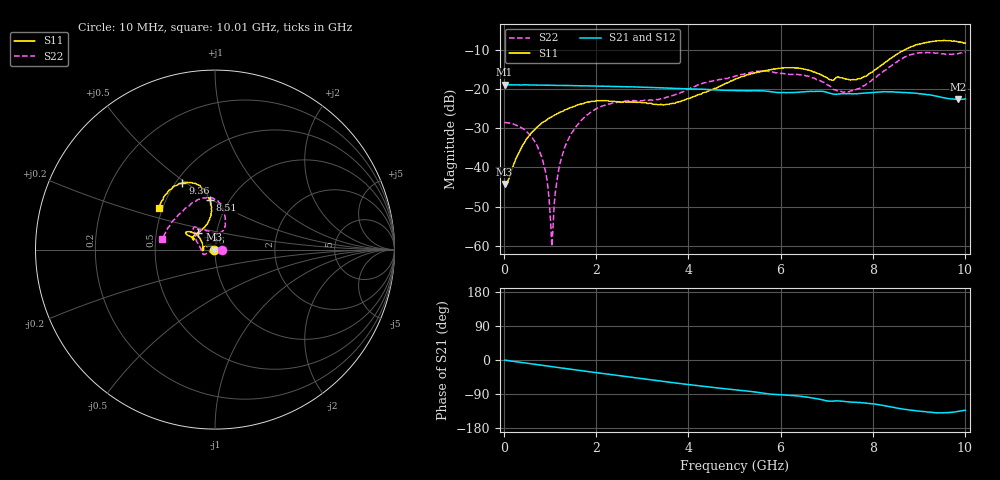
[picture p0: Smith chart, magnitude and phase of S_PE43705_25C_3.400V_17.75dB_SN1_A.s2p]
! Device ID: PE43705
! Serial: 1
! Insertion: A
! Impedance: 50 ohm
! Temp: 25C
! VDD: 3.400V
! Attenuation Step: 17.75dB
#  Hz  S  RI  R  50
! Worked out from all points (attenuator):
!   401 points, 10 MHz to 10.01 GHz, reference 50 ohm
!   highest |S21| = -18.83 dB at 10 MHz (marker M1); lowest = -22.6 dB at 9.86 GHz (marker M2)
!   lowest |S11| = -44.2 dB at 10 MHz (marker M3), VSWR 1.01, Z = 49.4 + j0.0483 ohm
!   |S11| at or under -10 dB: start of sweep to 8.677 GHz
!   |S22| runs from -60.1 to -10.4 dB; largest |S21 - S12| = 0.0014
!   S11 on the Smith chart (normalised r, x): 10 MHz: 0.99, +0.00; 7.46 GHz: 0.81, +0.16; 8.51 GHz: 0.82, +0.48; 9.36 GHz: 0.54, +0.48; 10.01 GHz: 0.48, +0.26
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1e7  -0.00614 0.000489  0.1144 -0.000478  0.1145 -0.000386  0.0375 -7.58e-06
4.1e8  -0.0103 0.0165  0.1132 -0.0135  0.1129 -0.0141  0.0309 0.00518
7.1e8  -0.0211 0.0248  0.1106 -0.0238  0.1106 -0.0237  0.0184 0.00594
8.85e8  -0.0292 0.026  0.1089 -0.0295  0.1089 -0.0293  0.0088 0.00354
1.01e9  -0.0349 0.0264  0.1074 -0.0333  0.1074 -0.0332  0.0015 0.00123
1.035e9  -0.0359 0.0263  0.1071 -0.0341  0.1071 -0.0339  4.8e-05 0.000984
1.085e9  -0.0383 0.026  0.1064 -0.0354  0.1064 -0.0354  -0.00328 -0.000315
1.16e9  -0.0416 0.0256  0.1056 -0.0376  0.1056 -0.0375  -0.00746 -0.00181
1.26e9  -0.0458 0.0243  0.1042 -0.0406  0.1043 -0.0405  -0.0135 -0.0041
1.435e9  -0.054 0.0215  0.1016 -0.0456  0.1017 -0.0456  -0.0243 -0.00857
1.685e9  -0.063 0.0156  0.0975 -0.0524  0.0975 -0.0524  -0.0378 -0.0153
2.26e9  -0.0708 -0.00113  0.0863 -0.0666  0.0864 -0.0666  -0.0585 -0.0276
3.36e9  -0.0634 0.00185  0.0596 -0.0857  0.0597 -0.0857  -0.0741 -0.00378
5.01e9  -0.1044 0.0843  0.0189 -0.0943  0.019 -0.0944  -0.1135 0.094
5.985e9  -0.1571 0.0993  -0.00246 -0.0906  -0.00214 -0.0905  -0.1038 0.1209
6.685e9  -0.1494 0.0786  -0.0167 -0.0922  -0.0168 -0.0923  -0.085 0.1119
7.46e9  -0.0952 0.0946  -0.0305 -0.0826  -0.0302 -0.0822  0.0111 0.0922
8.36e9  -0.0196 0.2402  -0.0506 -0.078  -0.0504 -0.078  0.0559 0.1844
8.51e9  -0.0284 0.2746  -0.0547 -0.0739  -0.0542 -0.0743  0.0482 0.215
9.36e9  -0.1812 0.3698  -0.062 -0.0535  -0.0619 -0.0536  -0.1125 0.2666
9.86e9  -0.2886 0.2788  -0.0529 -0.0518  -0.0528 -0.0511  -0.2557 0.1282
1.001e10  -0.3133 0.2311  -0.0511 -0.0553  -0.0519 -0.0555  -0.2939 0.0617
